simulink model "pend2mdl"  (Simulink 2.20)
settings: Solver=ode45  StartTime=0.0  StopTime=4.0  RelTol=1e-6  AbsTol=1e-6
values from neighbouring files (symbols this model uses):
  alpha = m*L/(J+m*L^2)    (= 2)    [PENDOL2.M]    (also in PENDOLO.M)
  Ao = beta1    (= -10)    [PENDOL2.M]
  Bo = [-alpha/M alpha*g-beta1^2]    [PENDOL2.M]
  Co = [0; 1]    [PENDOL2.M]
  Do = [0 1 ; 0 -beta1]    [PENDOL2.M]
  g = 9.81    [PENDOL2.M]    (also in PENDOLO.M)
  K = M*[alpha*g+lam1*lam2 -(lam1+lam2)]/alpha    [PENDOL2.M]    (also in PENDOLO.M)
  M = 2    [PENDOL2.M]    (also in PENDOLO.M)
  thdot0 = th00    (= 0.1)    [PENDOL2.M]    (also in PENDOLO.M = 1)
undefined symbols (not defined in the file or in its folder): th0
libraries: simulink x1

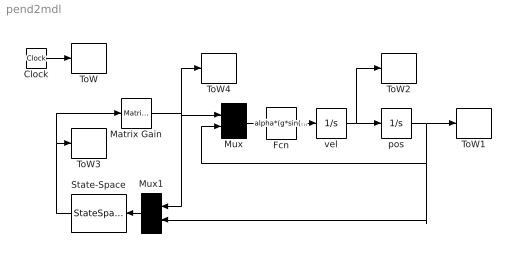
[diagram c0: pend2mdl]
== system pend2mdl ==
  Clock : Clock
  Fcn : Fcn  Expr=alpha*(g*sin(u(2))-u(1)*cos(u(2))/M)
  Matrix Gain : simulink/Linear/Matrix Gain  K=K
  Mux : Mux  Inputs=2
  Mux1 : Mux  Orientation=left  Inputs=2
  State-Space : StateSpace  Orientation=left  A=Ao  B=Bo  C=Co  D=Do  X0=0
  ToW : ToWorkspace  VariableName=t  SampleTime=-1
  ToW1 : ToWorkspace  VariableName=th  SampleTime=-1
  ToW2 : ToWorkspace  VariableName=thdot  SampleTime=-1
  ToW3 : ToWorkspace  VariableName=xtld  SampleTime=-1
  ToW4 : ToWorkspace  VariableName=u  SampleTime=-1
  pos : Integrator  ExternalReset=none  InitialConditionSource=internal  InitialCondition=th0  LimitOutput=off  UpperSaturationLimit=inf  LowerSaturationLimit=-inf  ShowSaturationPort=off  ShowStatePort=off  AbsoluteTolerance=auto
  vel : Integrator  ExternalReset=none  InitialConditionSource=internal  InitialCondition=thdot0  LimitOutput=off  UpperSaturationLimit=inf  LowerSaturationLimit=-inf  ShowSaturationPort=off  ShowStatePort=off  AbsoluteTolerance=auto
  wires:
  vel/1 -> pos/1, ToW2/1
  Matrix Gain/1 -> Mux/1, ToW4/1, Mux1/1
  Clock/1 -> ToW/1
  pos/1 -> ToW1/1, Mux1/2, Mux/2
  Fcn/1 -> vel/1
  Mux/1 -> Fcn/1
  Mux1/1 -> State-Space/1
  State-Space/1 -> Matrix Gain/1, ToW3/1
